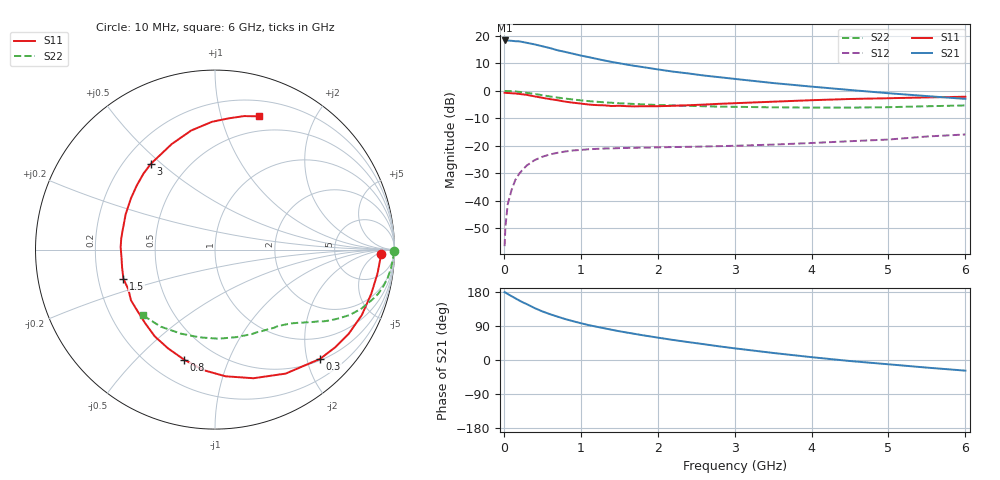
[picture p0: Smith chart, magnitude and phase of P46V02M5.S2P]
! SIEMENS Small Signal Semiconductors
! BFP182
! Si NPN RF Bipolar Junction Transistor in SOT143
! VCE = 6 V  IC = 2.5 mA
! Common Emitter S-Parameters:  March  1996
# GHz  S  MA  R  50
!  f  S11  S21  S12  S22
! GHz  MAG  ANG  MAG  ANG  MAG  ANG  MAG  ANG
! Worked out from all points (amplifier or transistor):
!   36 points, 10 MHz to 6 GHz, reference 50 ohm
!   highest |S21| = 18.3 dB at 10 MHz (marker M1)
!   |S21| within 3 dB of that: start of sweep to 628.4 MHz
!   unconditionally stable (mu >= 1): 2.08 GHz to 5.909 GHz
!   at 250 MHz: K = 0.14, MSG = 23.1 dB, |S12| = -28.5 dB
!   at 1.4 GHz: K = 0.73, MSG = 15.7 dB, |S12| = -20.9 dB
!   at 6 GHz: K = 0.99, MSG = 6.5 dB, |S12| = -15.8 dB
!   S11 on the Smith chart (normalised r, x): 10 MHz: 23, -7; 300 MHz: 0.53, -2.25; 800 MHz: 0.34, -0.70; 1.5 GHz: 0.31, -0.14; 3 GHz: 0.31, +0.46; 6 GHz: 0.35, +1.33
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0.01  0.9235 -1.5  8.257 178.9  0.0015 87.7  0.9946 -0.6
0.02  0.9226 -3.2  8.23 178.2  0.0033 86.2  0.9966 -1.3
0.05  0.9152 -8.3  8.237 174.2  0.0086 87.8  0.9926 -3.1
0.1  0.9049 -15.8  8.136 168.5  0.0157 80.4  0.9848 -6.4
0.2  0.8805 -32.1  7.952 157.1  0.0312 72.2  0.9598 -12.3
0.25  0.8629 -39.1  7.712 151.8  0.0376 67.5  0.9418 -15.2
0.3  0.8447 -46.1  7.471 147.3  0.0442 64.2  0.9198 -17.6
0.4  0.7952 -60.3  7.006 137.0  0.0551 56.9  0.879 -22.0
0.5  0.7482 -73.3  6.48 128.3  0.0633 50.6  0.8342 -25.9
0.6  0.7085 -85.2  6.003 120.9  0.07 45.4  0.7914 -28.9
0.7  0.6746 -95.5  5.466 114.3  0.0749 41.2  0.7558 -31.4
0.8  0.6364 -105.8  5.1 107.9  0.0791 37.4  0.7245 -33.5
1  0.5885 -124.8  4.388 97.1  0.0843 31.6  0.6729 -36.9
1.1  0.5651 -133.6  4.117 92.2  0.0867 29.4  0.652 -38.4
1.5  0.5358 -162.4  3.179 75.9  0.091 23.3  0.596 -43.5
1.8  0.5259 178.3  2.717 65.5  0.093 21.0  0.5695 -47.3
2.2  0.5353 158.3  2.238 52.9  0.0952 19.0  0.5456 -53.0
3  0.5968 126.8  1.652 30.8  0.1004 18.5  0.5133 -66.5
3.5  0.6356 112.3  1.389 18.6  0.1055 18.7  0.502 -76.4
4.5  0.7121 91.4  1.038 -2.7  0.1215 19.3  0.4964 -99.9
5.5  0.761 77.8  0.804 -20.1  0.148 18.1  0.5252 -125.2
6  0.7822 71.7  0.715 -28.1  0.1613 15.0  0.5435 -137.7
